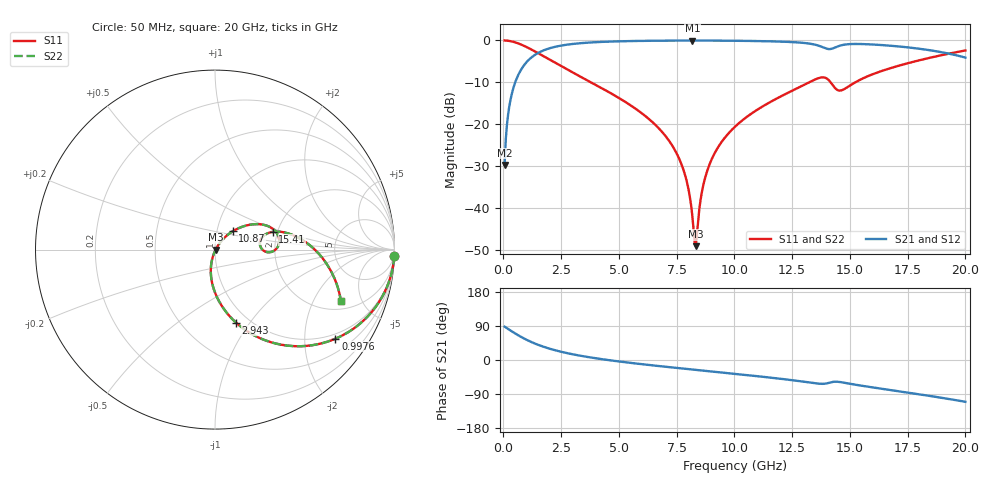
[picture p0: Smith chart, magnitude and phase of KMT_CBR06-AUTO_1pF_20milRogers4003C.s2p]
! Data measured by Modelithics Inc. support@modelithics.com 813-866-6335
! KEMET CBR06-AUTO 1pF, Pad Width= 0.851mm, Pad Length= 0.64mm, Pad Gap= 0.62mm, 20mil Rogers 4003C substrate Data, January 2022
# hz S ma R 50
! 2 Port Network Data from SP1.SP block
! freq  magS11  angS11  magS21  angS21  magS12  angS12  magS22  angS22
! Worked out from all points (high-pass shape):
!   401 points, 50 MHz to 20 GHz, reference 50 ohm
!   highest |S21| = -0.03 dB at 8.18 GHz (marker M1); lowest = -29.7 dB at 50 MHz (marker M2)
!   |S21| within 3 dB of the highest: 1.49 GHz to 19.18 GHz (17.69 GHz wide, 171 % of centre)
!   lowest |S11| = -49.1 dB at 8.329 GHz (marker M3), VSWR 1.01, Z = 50.3 - j0.0671 ohm
!   |S11| at or under -10 dB: 3.789 GHz to 13.24 GHz (9.447 GHz wide, 111 % of centre); 14.17 GHz to 15.23 GHz (1.069 GHz wide, 7.27 % of centre)
!   |S22| runs from -49.1 to 0.0 dB; largest |S21 - S12| = 0
!   S11 on the Smith chart (normalised r, x): 50 MHz: 1, -57; 997.6 MHz: 0.86, -2.80; 2.943 GHz: 0.87, -0.86; 10.87 GHz: 1.19, +0.25; 15.41 GHz: 1.89, +0.42; 20 GHz: 2.46, -3.35
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5e7  0.9995 -2.0  0.03259 88.0  0.03259 88.0  0.9995 -2.0
2.495e8  0.9869 -10.0  0.1607 79.9  0.1607 79.9  0.9869 -10.0
3.99125e8  0.9675 -15.9  0.2523 74.1  0.2523 74.1  0.9675 -15.9
9.97625e8  0.8348 -36.5  0.5495 53.5  0.5495 53.5  0.8348 -36.5
1.895375e9  0.6118 -58.1  0.7894 31.7  0.7894 31.7  0.6118 -58.1
2.94275e9  0.4226 -74.0  0.9042 15.7  0.9042 15.7  0.4226 -74.0
3.391625e9  0.3623 -79.1  0.9298 10.6  0.9298 10.6  0.3623 -79.1
6.73325e9  0.08871 -104.1  0.9929 -16.0  0.9929 -16.0  0.08871 -104.1
7.73075e9  0.03191 -106.6  0.996 -22.4  0.996 -22.4  0.03191 -106.6
7.980125e9  0.01835 -103.7  0.9963 -23.9  0.9963 -23.9  0.01835 -103.7
8.179625e9  0.007928 -90.4  0.9964 -25.1  0.9964 -25.1  0.007928 -90.4
8.32925e9  0.003488 -11.0  0.9963 -26.1  0.9963 -26.1  0.003488 -11.0
8.6285e9  0.01741 50.6  0.9961 -27.9  0.9961 -27.9  0.01741 50.6
8.877875e9  0.0307 53.9  0.9956 -29.4  0.9956 -29.4  0.0307 53.9
1.0025e10  0.09316 50.8  0.9911 -36.5  0.9911 -36.5  0.09316 50.8
1.087288e10  0.1418 46.0  0.9844 -41.9  0.9844 -41.9  0.1418 46.0
1.336662e10  0.3291 22.7  0.9051 -60.4  0.9051 -60.4  0.3291 22.7
1.42145e10  0.3035 -2.8  0.796 -58.4  0.796 -58.4  0.3035 -2.8
1.46135e10  0.2528 8.5  0.8733 -58.5  0.8733 -58.5  0.2528 8.5
1.54115e10  0.336 17.1  0.9071 -67.0  0.9071 -67.0  0.336 17.1
1.670825e10  0.4621 8.8  0.8668 -78.8  0.8668 -78.8  0.4621 8.8
2e10  0.7589 -22.3  0.6236 -110.3  0.6236 -110.3  0.7589 -22.3
